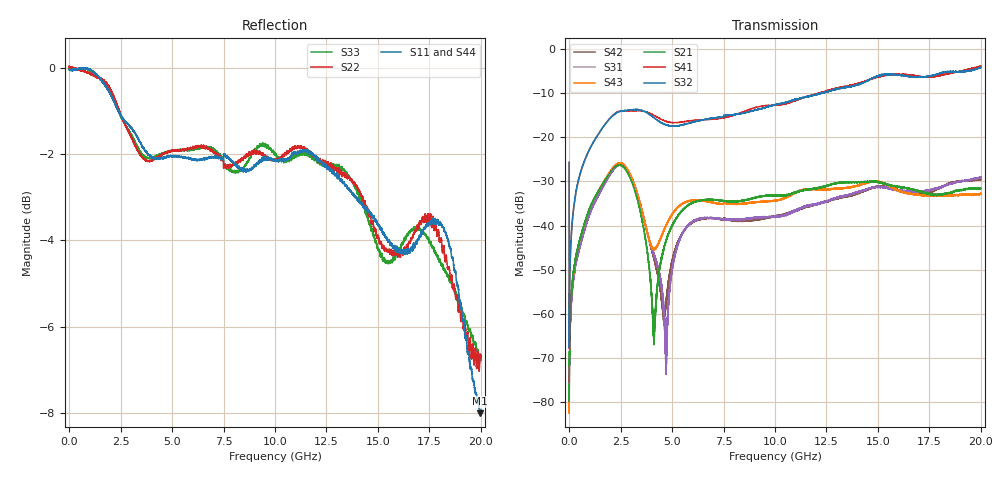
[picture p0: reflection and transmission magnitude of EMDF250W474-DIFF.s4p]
!EMDF250W474
!Johanson Technology Inc.
!www.johansontechnology.com
!Test Board Conditions:
!Substrate Type  RO4350B
!Substrate Thickness  21 mil
!Substrate Dk  3.66
!TL Type: GCPW
!TL Trace Width  40 mil
!TL Gap  17.5 mil
!PART MODE DIFFERENTIAL
!DUT TOPOLOGY	DIFFERENTIAL 4-PORT
# MHz S  dB  R 50
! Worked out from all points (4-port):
!   20001 points, 300 kHz to 20 GHz, reference 50 ohm
!   strongest paths, dB at 300 kHz, 5 GHz, 10 GHz, 15 GHz, 20 GHz:
!     S32: -25.7, -17.5, -12.7, -6.2, -4.2
!     S41: -25.7, -16.7, -12.8, -6.4, -4.0
!     S21: -75.9, -40.1, -33.3, -30.2, -31.6
!     S43: -73.9, -37.4, -34.3, -30.1, -32.7
!     S31: -72.6, -50.2, -38.0, -31.3, -29.0
!     S42: -72.0, -48.1, -37.9, -31.2, -29.6
!   lowest |S11| = -8.0 dB at 19.96 GHz (marker M1), VSWR 2.32, Z = 26.5 - j21 ohm
!   |S11| at or under -10 dB: nowhere
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0.3  -0.04 -176.9  -68.41 -22.3  -93.83 -102.7  -25.69 -86.0
     -75.92 -63.0  0.03 -177.0  -25.77 -86.3  -75.04 -39.1
     -72.59 -85.2  -25.70 -86.1  -0.05 -176.9  -68.28 -74.3
     -25.72 -86.0  -72.00 -26.0  -73.95 -30.9  0.08 -176.8
2399.264  -1.02 138.4  -26.30 -19.5  -26.36 -25.6  -14.14 23.0
          -26.34 -19.3  -0.95 140.5  -14.33 25.1  -26.26 -26.5
          -26.37 -25.7  -14.31 24.9  -1.01 141.5  -25.80 -22.1
          -14.18 23.2  -26.27 -26.7  -25.82 -21.9  -1.05 141.1
4113.238  -2.10 122.1  -65.55 136.0  -46.49 -133.6  -14.99 -26.2
          -66.33 146.2  -2.12 125.5  -15.57 -29.4  -47.39 -151.1
          -46.34 -133.4  -15.57 -29.4  -2.08 129.0  -45.08 134.2
          -15.03 -26.0  -47.21 -150.5  -45.35 134.3  -2.00 127.2
4706.229  -2.08 119.4  -43.50 42.4  -69.08 109.1  -16.42 -31.3
          -43.50 42.2  -1.97 117.7  -17.23 -30.8  -58.10 80.5
          -69.09 145.8  -17.23 -31.1  -1.98 122.0  -39.92 66.0
          -16.43 -30.9  -56.71 83.3  -39.99 67.0  -2.01 121.2
6107.208  -2.15 97.7  -34.51 -5.6  -38.86 -31.2  -16.08 -34.3
          -34.58 -5.9  -1.84 102.5  -16.54 -29.5  -38.96 -27.9
          -38.79 -31.1  -16.47 -29.2  -1.89 102.4  -34.15 -5.5
          -16.20 -34.8  -38.88 -27.6  -34.30 -6.0  -1.85 102.5
19962  -8.01 -122.8  -31.80 57.1  -29.17 37.6  -4.26 138.6
       -31.56 56.3  -6.72 -114.6  -4.05 144.2  -29.65 42.6
       -29.04 38.1  -4.28 145.0  -6.72 -101.5  -33.21 68.1
       -4.00 137.6  -29.60 42.2  -32.84 67.1  -6.86 -99.7
20000  -7.94 -124.5  -31.66 56.3  -29.14 36.6  -4.18 137.7
       -31.60 54.5  -6.71 -112.7  -4.06 144.1  -29.67 41.9
       -29.01 36.1  -4.23 144.6  -6.77 -101.9  -33.20 67.1
       -3.97 136.8  -29.59 41.8  -32.74 66.2  -6.92 -99.9
